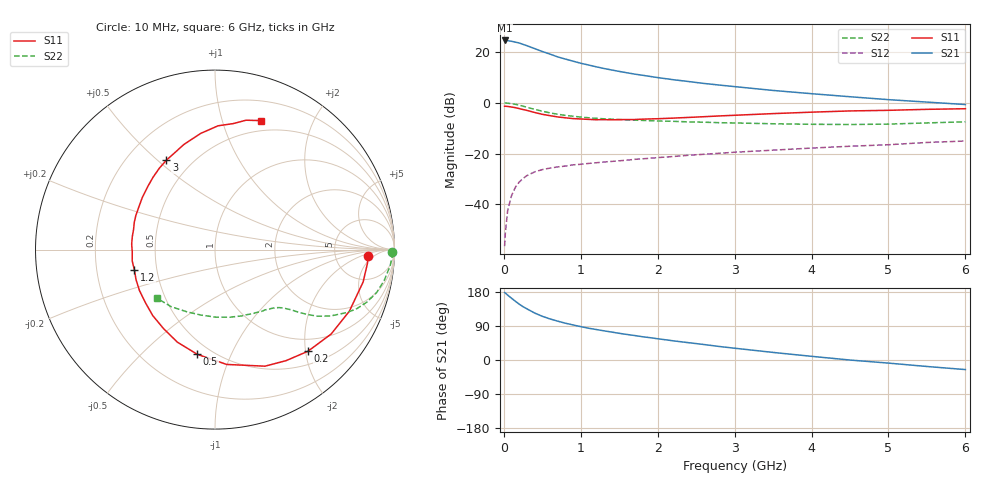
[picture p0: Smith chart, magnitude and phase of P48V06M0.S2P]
! SIEMENS Small Signal Semiconductors
! BFP182
! Si NPN RF Bipolar Junction Transistor in SOT143
! VCE = 8 V  IC = 6 mA
! Common Emitter S-Parameters:  March  1996
# GHz  S  MA  R  50
!  f  S11  S21  S12  S22
! GHz  MAG  ANG  MAG  ANG  MAG  ANG  MAG  ANG
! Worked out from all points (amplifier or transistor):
!   36 points, 10 MHz to 6 GHz, reference 50 ohm
!   highest |S21| = 24.5 dB at 10 MHz (marker M1)
!   |S21| within 3 dB of that: start of sweep to 382.2 MHz
!   unconditionally stable (mu >= 1): 1.552 GHz to 5.66 GHz
!   at 250 MHz: K = 0.23, MSG = 26.4 dB, |S12| = -29.8 dB
!   at 1.4 GHz: K = 0.95, MSG = 18.0 dB, |S12| = -23.1 dB
!   at 6 GHz: K = 0.97, MSG = 7.2 dB, |S12| = -15.1 dB
!   lowest NFmin = 1.25 dB at 450 MHz
!   S11 on the Smith chart (normalised r, x): 10 MHz: 12, -3; 200 MHz: 0.74, -2.05; 500 MHz: 0.42, -0.75; 1.2 GHz: 0.37, -0.11; 3 GHz: 0.36, +0.53; 6 GHz: 0.39, +1.34
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0.01  0.8527 -2.3  16.84 178.0  0.0015 82.1  0.9879 -0.9
0.05  0.8449 -12.3  16.69 171.2  0.0076 85.5  0.9802 -5.2
0.1  0.8236 -24.6  16.23 163.0  0.0148 75.7  0.9585 -10.3
0.15  0.8001 -36.0  15.61 155.0  0.0217 69.9  0.9318 -14.9
0.2  0.7673 -47.6  15.01 147.3  0.0274 65.6  0.8951 -19.1
0.25  0.7345 -57.4  14.1 140.7  0.0323 61.2  0.8551 -22.7
0.3  0.7067 -66.8  13.27 135.0  0.0368 57.0  0.8142 -25.5
0.4  0.6431 -84.2  11.65 124.0  0.0435 51.4  0.7422 -29.9
0.5  0.5918 -99.6  10.2 115.3  0.0483 46.2  0.6813 -33.0
0.6  0.5567 -112.1  9.071 108.4  0.0517 43.7  0.6313 -35.0
0.7  0.5256 -123.0  7.99 102.5  0.0545 41.3  0.5934 -36.4
0.8  0.5053 -133.4  7.243 97.1  0.0567 39.5  0.5639 -37.5
1  0.4787 -151.6  5.99 88.0  0.0614 37.3  0.5223 -39.3
1.1  0.4707 -159.2  5.536 83.9  0.0638 37.4  0.5064 -40.2
1.2  0.463 -165.9  5.103 80.5  0.0658 36.6  0.4935 -41.1
1.6  0.4664 171.2  3.891 67.4  0.074 36.0  0.46 -45.1
2.2  0.4983 144.4  2.846 50.7  0.0873 35.1  0.431 -53.1
3  0.5667 118.6  2.078 31.1  0.1061 32.1  0.3999 -67.2
3.5  0.6112 106.4  1.747 20.0  0.1165 29.3  0.3856 -77.6
4.5  0.6899 88.6  1.313 -0.1  0.1391 23.9  0.3729 -101.9
5.5  0.7414 76.5  1.03 -17.1  0.1652 18.4  0.4007 -127.3
6  0.7624 70.5  0.922 -25.3  0.1763 14.2  0.4213 -139.8
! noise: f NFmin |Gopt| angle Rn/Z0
0.45  1.25  0.25  39  0.3
0.9  1.4  0.25  78  0.23
1.8  1.95  0.21  151  0.2
